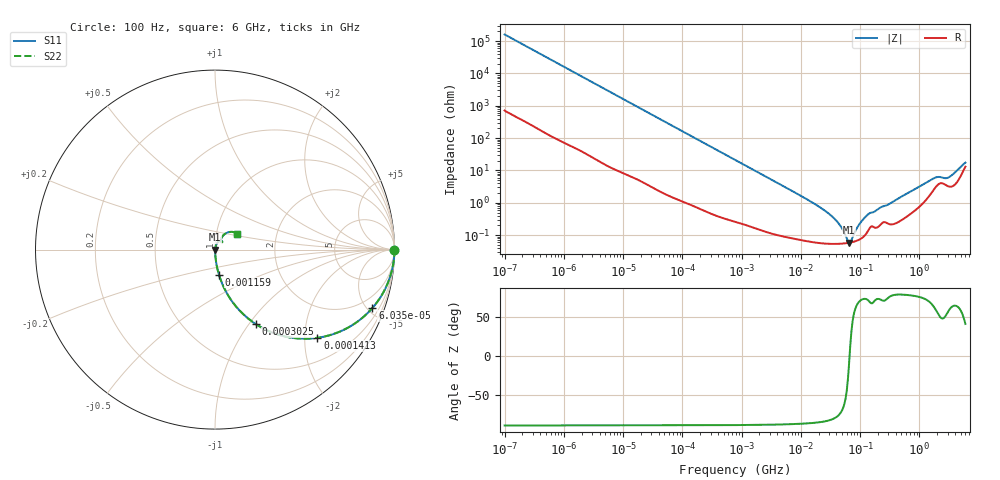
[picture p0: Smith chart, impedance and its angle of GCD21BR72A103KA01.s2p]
!Murata Part Number: GCD21BR72A103KA01
!These Parameters are Measured in Series Mode Connection
!Data Generated on Mar 13, 2026
!  o--ll--o
!Port1  Port2
!  o------o
!Operation Temp=25[degC], DC Bias Voltage=0[V]
!Freq. Start=100[Hz] Stop=6[GHz] 401[Steps]
# Hz S RI R 50
!Freq.(Hz) S11(Real) S11(Imag) S21(Real) S21(Imag) S12(Real) S12(Imag) S22(Real) S22(Imag)
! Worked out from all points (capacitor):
!   401 points, 100 Hz to 6 GHz, reference 50 ohm
!   read as one part in series: C = 9.97 nF near 109 Hz
!   lowest |Z| = 59 mohm at 65.19 MHz (marker M1)
!   series resonance near 66.55 MHz, so ESL is about 570 pH
!   S11 on the Smith chart (normalised r, x): 100 Hz: open; 60.35 kHz: 1.03, -5.38; 141.3 kHz: 1.02, -2.31; 302.5 kHz: 1.01, -1.08; 1.159 MHz: 1.00, -0.28; 6 GHz: 1.26, +0.23
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100  1 -0.000627  3.2e-06 0.000627  3.2e-06 0.000627  1 -0.000627
2008  0.9998 -0.0125  0.000216 0.0125  0.000216 0.0125  0.9998 -0.0125
12041  0.9941 -0.0741  0.00591 0.0741  0.00591 0.0741  0.9941 -0.0741
40335  0.9406 -0.2334  0.0594 0.2334  0.0594 0.2334  0.9406 -0.2334
60352  0.8773 -0.3251  0.1227 0.3251  0.1227 0.3251  0.8773 -0.3251
141303  0.5705 -0.4913  0.4295 0.4913  0.4295 0.4913  0.5705 -0.4913
302498  0.2282 -0.4154  0.7718 0.4154  0.7718 0.4154  0.2282 -0.4154
774597  0.0453 -0.202  0.9547 0.202  0.9547 0.202  0.0453 -0.202
1159002  0.0218 -0.1388  0.9782 0.1388  0.9782 0.1388  0.0218 -0.1388
3245845  0.0037 -0.0508  0.9963 0.0508  0.9963 0.0508  0.0037 -0.0508
1.555665e7  0.000714 -0.0102  0.9993 0.0102  0.9993 0.0102  0.000714 -0.0102
3.80911e7  0.000544 -0.003  0.9995 0.003  0.9995 0.003  0.000544 -0.003
4.764863e7  0.000546 -0.00174  0.9995 0.00174  0.9995 0.00174  0.000546 -0.00174
5.960426e7  0.000566 -0.000567  0.9994 0.000567  0.9994 0.000567  0.000566 -0.000567
6.518806e7  0.00058 -0.000106  0.9994 0.000106  0.9994 0.000106  0.00058 -0.000106
7.129496e7  0.000599 0.000358  0.9994 -0.000358  0.9994 -0.000358  0.000599 0.000358
9.326766e7  0.000705 0.0018  0.9993 -0.0018  0.9993 -0.0018  0.000705 0.0018
1.275994e8  0.00113 0.00375  0.9989 -0.00375  0.9989 -0.00375  0.00113 0.00375
3.124326e8  0.00226 0.00893  0.9977 -0.00893  0.9977 -0.00893  0.00226 0.00893
1.712697e9  0.0256 0.048  0.9744 -0.048  0.9744 -0.048  0.0256 0.048
3.205649e9  0.0333 0.0506  0.9667 -0.0506  0.9667 -0.0506  0.0333 0.0506
6e9  0.1245 0.0889  0.8755 -0.0889  0.8755 -0.0889  0.1245 0.0889
